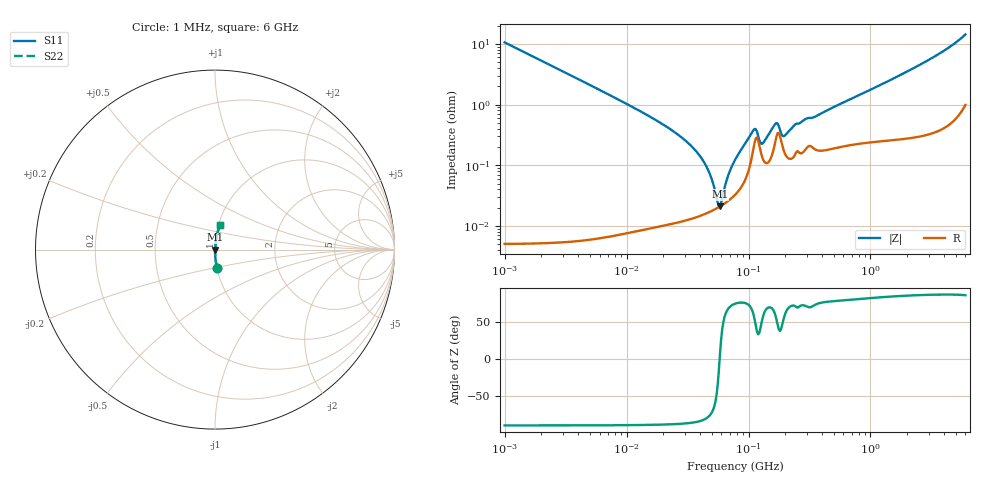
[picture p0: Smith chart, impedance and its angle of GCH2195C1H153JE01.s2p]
!Murata Part Number: GCH2195C1H153JE01
!These Parameters are Measured in Series Mode Connection
!Data Generated on Mar 13, 2026
!  o--ll--o
!Port1  Port2
!  o------o
!Operation Temp=25[degC], DC Bias Voltage=0[V]
!Freq. Start=1000[kHz] Stop=6[GHz] 401[Steps]
# Hz S RI R 50
!Freq.(Hz) S11(Real) S11(Imag) S21(Real) S21(Imag) S12(Real) S12(Imag) S22(Real) S22(Imag)
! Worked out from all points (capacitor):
!   401 points, 1 MHz to 6 GHz, reference 50 ohm
!   read as one part in series: C = 15 nF near 1.044 MHz
!   lowest |Z| = 21.1 mohm at 58.38 MHz (marker M1)
!   series resonance near 57.98 MHz, so ESL is about 500 pH
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1000000  0.0112 -0.105  0.9888 0.105  0.9888 0.105  0.0112 -0.105
4293785  0.000661 -0.0246  0.9993 0.0246  0.9993 0.0246  0.000661 -0.0246
1.843659e7  0.000124 -0.00517  0.9999 0.00517  0.9999 0.00517  0.000124 -0.00517
2.910942e7  0.000127 -0.00274  0.9999 0.00274  0.9999 0.00274  0.000127 -0.00274
3.947016e7  0.000147 -0.00146  0.9999 0.00146  0.9999 0.00146  0.000147 -0.00146
4.697123e7  0.000167 -0.000793  0.9998 0.000793  0.9998 0.000793  0.000167 -0.000793
5.013812e7  0.000177 -0.000547  0.9998 0.000547  0.9998 0.000547  0.000177 -0.000547
5.589783e7  0.000199 -0.000138  0.9998 0.000138  0.9998 0.000138  0.000199 -0.000138
5.838291e7  0.000209 2.68e-05  0.9998 -2.68e-05  0.9998 -2.68e-05  0.000209 2.68e-05
6.798347e7  0.000258 0.000622  0.9997 -0.000622  0.9997 -0.000622  0.000258 0.000622
7.745967e7  0.000326 0.00118  0.9997 -0.00118  0.9997 -0.00118  0.000326 0.00118
1.096987e8  0.00189 0.00329  0.9981 -0.00329  0.9981 -0.00329  0.00189 0.00329
1.145757e8  0.00277 0.00279  0.9972 -0.00279  0.9972 -0.00279  0.00277 0.00279
1.249896e8  0.00178 0.00153  0.9982 -0.00153  0.9982 -0.00153  0.00178 0.00153
1.305463e8  0.0013 0.00188  0.9987 -0.00188  0.9987 -0.00188  0.0013 0.00188
1.658303e8  0.00246 0.00412  0.9975 -0.00412  0.9975 -0.00412  0.00246 0.00412
1.973453e8  0.00161 0.0026  0.9984 -0.0026  0.9984 -0.0026  0.00161 0.0026
2.400133e8  0.0015 0.00442  0.9985 -0.00442  0.9985 -0.00442  0.0015 0.00442
3.325952e8  0.00202 0.00571  0.998 -0.00571  0.998 -0.00571  0.00202 0.00571
1.428092e9  0.00316 0.0247  0.9968 -0.0247  0.9968 -0.0247  0.00316 0.0247
3.408564e9  0.00744 0.0626  0.9926 -0.0626  0.9926 -0.0626  0.00744 0.0626
6e9  0.0293 0.1376  0.9707 -0.1376  0.9707 -0.1376  0.0293 0.1376
